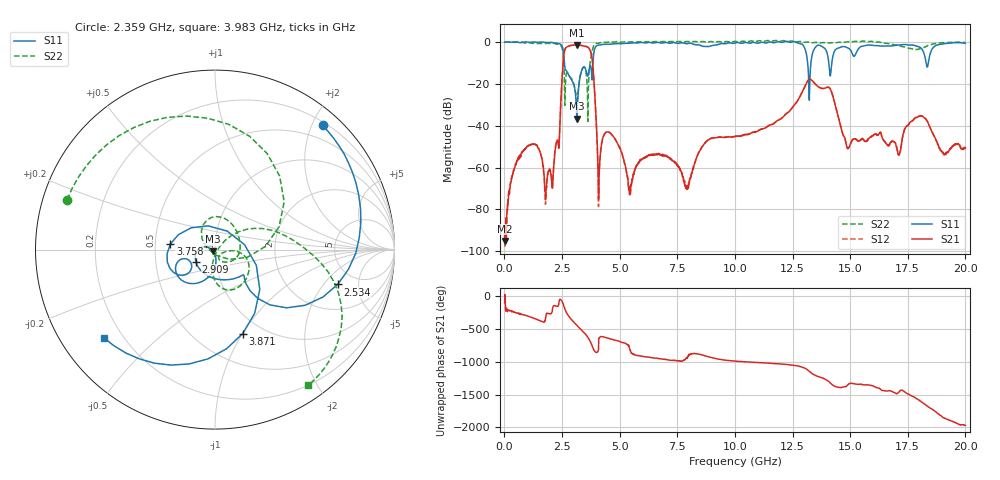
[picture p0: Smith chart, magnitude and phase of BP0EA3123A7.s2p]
! 9/17/2020 12:44:07 PM
! C:\ANRITSUVNA\DATA\MLO\SAMPLES\RAYTHEOM BP\17364_20GH_91720 .S2P
! CHANNEL.1
! TR.MEASUREMENT
! CORRECTED.DATA
# GHZ S RI R 50.0
! FREQ.GHZ  S11RE  S11IM  S31RE  S31IM  S13RE  S13IM  S33RE  S33IM
!; PortSelection: Port_13
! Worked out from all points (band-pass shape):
!   1601 points, 10 MHz to 20 GHz, reference 50 ohm
!   highest |S21| = -1.42 dB at 3.133 GHz (marker M1); lowest = -95.1 dB at 34.99 MHz (marker M2)
!   |S21| within 3 dB of the highest: 2.605 GHz to 3.734 GHz (1.129 GHz wide, 35.6 % of centre)
!   lowest |S11| = -36.7 dB at 3.146 GHz (marker M3), VSWR 1.03, Z = 48.8 - j0.849 ohm
!   |S11| at or under -10 dB: 2.605 GHz to 3.843 GHz (1.238 GHz wide, 38.4 % of centre); 13.16 GHz to 13.3 GHz (143 MHz wide, 1.08 % of centre); 14.07 GHz to 14.2 GHz (130.3 MHz wide, 0.921 % of centre)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
!   |S22| runs from -37.9 to 0.7 dB; largest |S21 - S12| = 0.0022
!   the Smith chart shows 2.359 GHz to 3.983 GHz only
!   S11 on the Smith chart (normalised r, x): 2.359 GHz: 0.25, +2.16; 2.534 GHz: 3.59, -2.82; 2.909 GHz: 0.80, -0.11; 3.758 GHz: 0.60, +0.04; 3.871 GHz: 0.81, -1.00; 3.983 GHz: 0.13, -0.34
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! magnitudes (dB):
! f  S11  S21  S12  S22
! 10 MHz  -0.1  -92.9  -87.6  0.0
! 34.99 MHz  -0.1  -95.1  -88.6  -0.1
! 1.059 GHz  -0.1  -49.6  -49.4  -0.4
! 1.834 GHz  -0.3  -67.3  -69.3  -0.7
! 2.359 GHz  -0.8  -50.7  -50.9  -1.2
! 2.534 GHz  -3.0  -12.2  -12.2  -4.3
! 2.909 GHz  -17.9  -1.6  -1.6  -17.4
! 3.133 GHz  -34.1  -1.4  -1.4  -27.1
! 3.146 GHz  -36.7  -1.4  -1.4  -27.7
! 3.346 GHz  -13.9  -1.7  -1.7  -13.8
! 3.758 GHz  -12.0  -5.2  -5.2  -7.1
! 3.871 GHz  -6.1  -16.0  -16.0  -1.9
! 3.983 GHz  -2.0  -37.7  -37.6  -0.8
! 4.12 GHz  -1.4  -60.4  -60.5  -0.5
! 5.432 GHz  -0.6  -73.1  -70.1  0.0
! 6.682 GHz  -0.3  -53.3  -53.7  0.0
! 7.919 GHz  -0.9  -70.4  -70.4  0.2
! 10.01 GHz  -0.5  -45.1  -45.1  0.2
! 13.34 GHz  -6.8  -18.4  -18.4  -0.4
! 14.9 GHz  -2.9  -50.8  -51.1  0.1
! 16.68 GHz  -2.0  -49.5  -49.2  -0.8
! 20 GHz  -0.7  -50.7  -50.4  -0.2
